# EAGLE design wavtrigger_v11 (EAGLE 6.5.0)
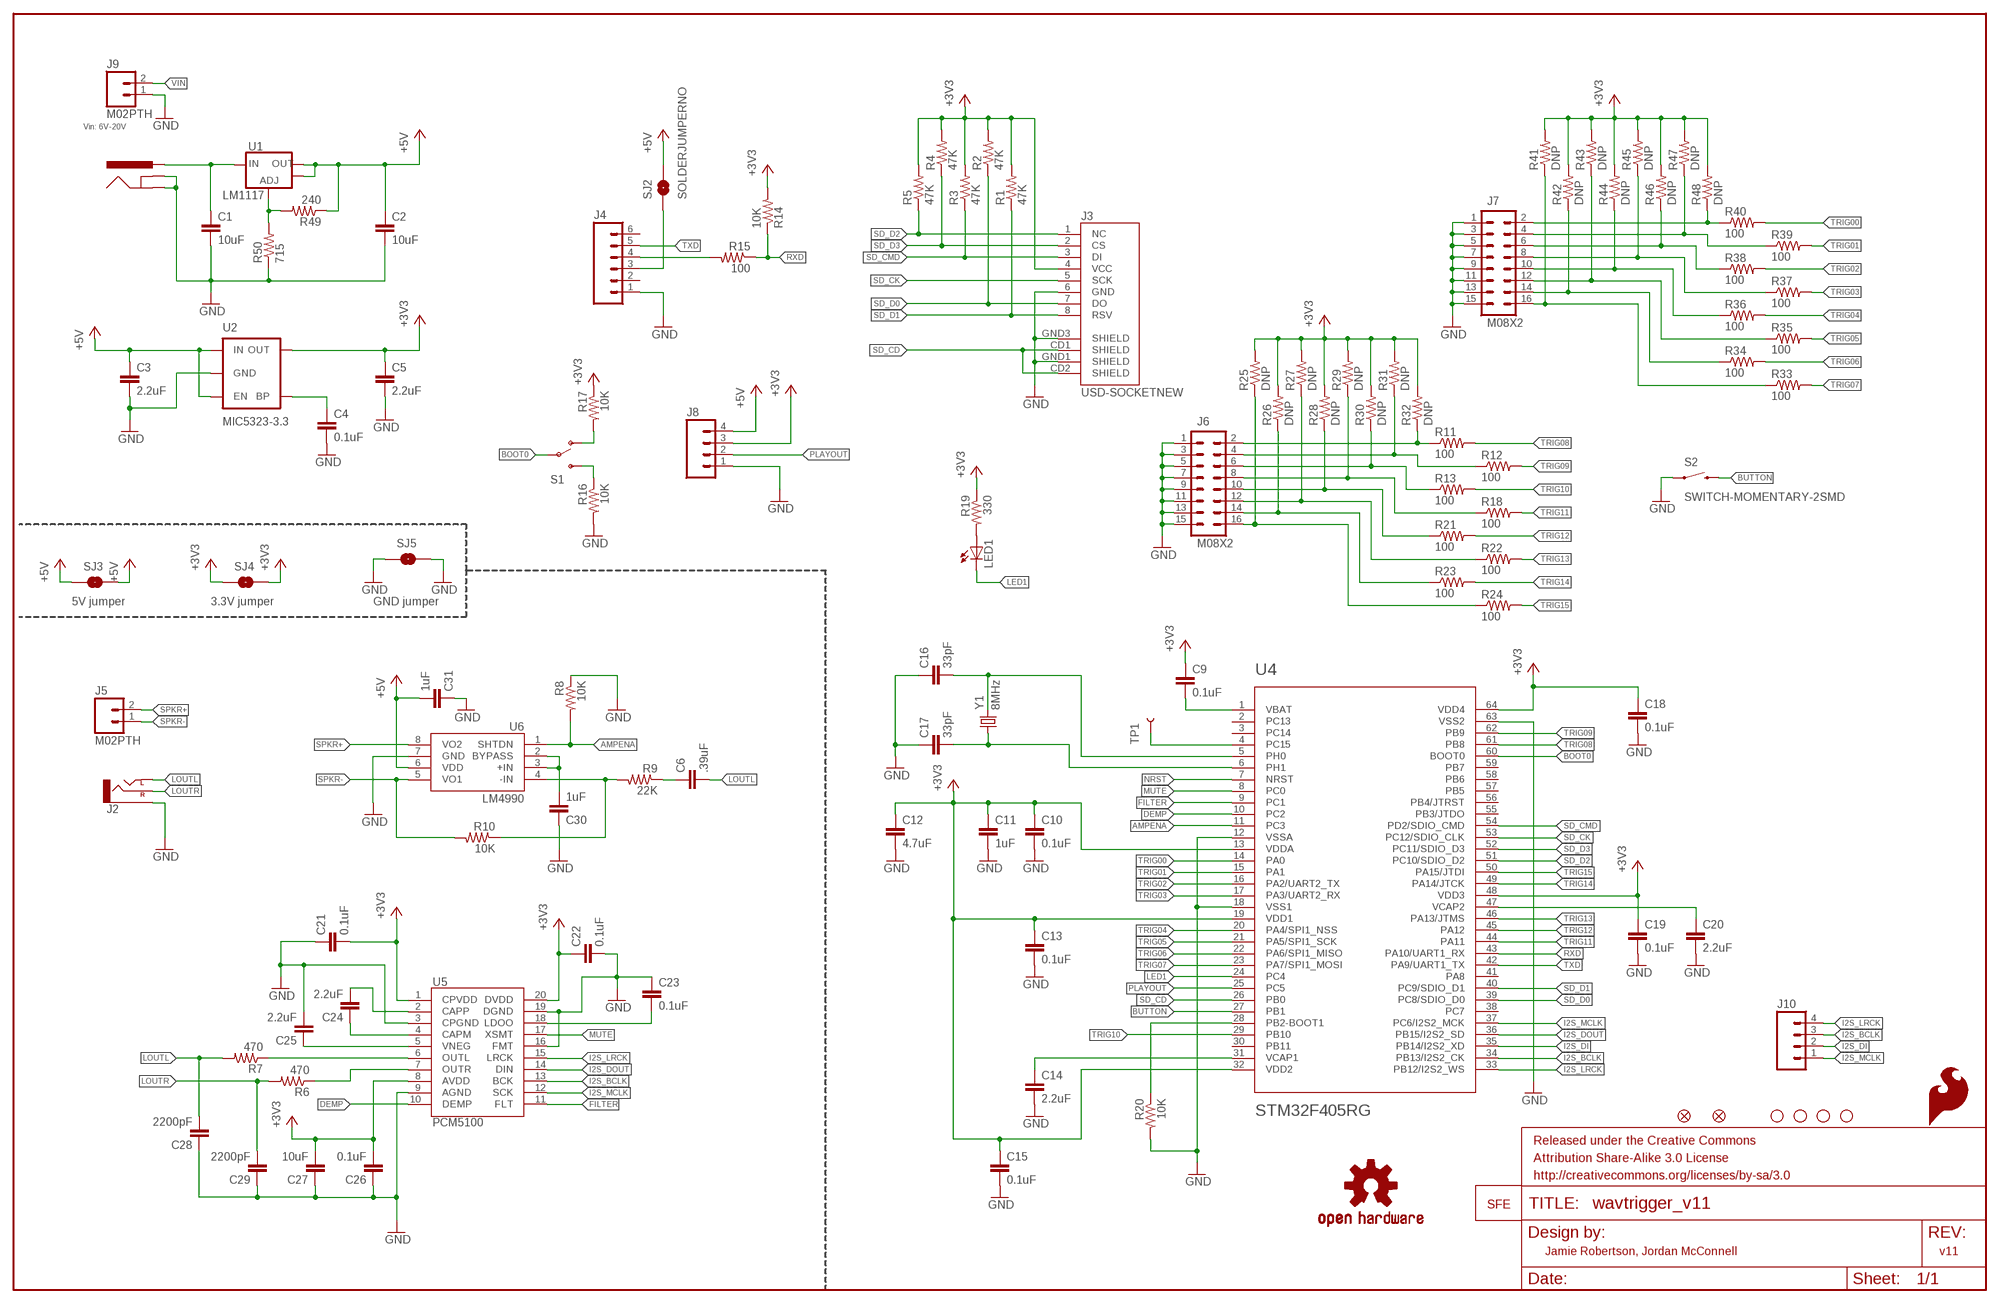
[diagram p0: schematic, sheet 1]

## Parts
C1  10uF  10UF50V20%(1210)  [1210]
C2  10uF  1UF-25V-10%(0805)  [0805]
C3  2.2uF  1UF-25V-10%(0805)  [0805]
C4  0.1uF  CAP0603-CAP  [0603-CAP]
C5  2.2uF  1UF-25V-10%(0805)  [0805]
C6  .39uF  CAP0603-CAP  [0603-CAP]
C9  0.1uF  CAP0603-CAP  [0603-CAP]
C10  0.1uF  CAP0603-CAP  [0603-CAP]
C11  1uF  CAP0603-CAP  [0603-CAP]
C12  4.7uF  CAP0603-CAP  [0603-CAP]
C13  0.1uF  CAP0603-CAP  [0603-CAP]
C14  2.2uF  CAP0603-CAP  [0603-CAP]
C15  0.1uF  CAP0603-CAP  [0603-CAP]
C16  33pF  CAP0603-CAP  [0603-CAP]
C17  33pF  CAP0603-CAP  [0603-CAP]
C18  0.1uF  CAP0603-CAP  [0603-CAP]
C19  0.1uF  CAP0603-CAP  [0603-CAP]
C20  2.2uF  CAP0603-CAP  [0603-CAP]
C21  0.1uF  CAP0603-CAP  [0603-CAP]
C22  0.1uF  CAP0603-CAP  [0603-CAP]
C23  0.1uF  CAP0603-CAP  [0603-CAP]
C24  2.2uF  CAP0603-CAP  [0603-CAP]
C25  2.2uF  CAP0603-CAP  [0603-CAP]
C26  0.1uF  CAP0603-CAP  [0603-CAP]
C27  10uF  CAP0603-CAP  [0603-CAP]
C28  2200pF  CAP0603-CAP  [0603-CAP]
C29  2200pF  CAP0603-CAP  [0603-CAP]
C30  1uF  CAP0603-CAP  [0603-CAP]
C31  1uF  CAP0603-CAP  [0603-CAP]
FID1  FIDUCIAL1X2  [FIDUCIAL-1X2]
FID2  FIDUCIAL1X2  [FIDUCIAL-1X2]
FRAME2  FRAME-LEDGER  [CREATIVE_COMMONS]
J1  5.5x2.1mm Barrel  POWER_JACKOVERPASTE_REDBOARD_0603  [POWER_JACK_SMD_OVERPASTE_REDBOARD_0603]
J2  AUDIO-JACKSMD2  [AUDIO-JACK-3.5MM-SMD]
J3  USD-SOCKETNEW  [MICRO-SD-SOCKET-PP]
J4  M06SIP  [1X06]
J5  M02PTH  [1X02]
J6  M08X2  [2X8]
J7  M08X2  [2X8]
J8  M04PTH  [1X04]
J9  M02PTH  [1X02]
J10  M04PTH  [1X04]
LED1  LED0603  [LED-0603]
LOGO1  OSHW-LOGOL  [OSHW-LOGO-L]
LOGO2  LOGO-SFENEW  [SFE-NEW-WEBLOGO]
LOGO4  SFE_LOGO_FLAME.2_INCH  [SFE_LOGO_FLAME_.2]
R1  47K  RESISTOR0603-RES  [0603-RES]
R2  47K  RESISTOR0603-RES  [0603-RES]
R3  47K  RESISTOR0603-RES  [0603-RES]
R4  47K  RESISTOR0603-RES  [0603-RES]
R5  47K  RESISTOR0603-RES  [0603-RES]
R6  470  RESISTOR0603-RES  [0603-RES]
R7  470  RESISTOR0603-RES  [0603-RES]
R8  10K  RESISTOR0603-RES  [0603-RES]
R9  22K  RESISTOR0603-RES  [0603-RES]
R10  10K  RESISTOR0603-RES  [0603-RES]
R11  100  RESISTOR0603-RES  [0603-RES]
R12  100  RESISTOR0603-RES  [0603-RES]
R13  100  RESISTOR0603-RES  [0603-RES]
R14  10K  RESISTOR0603-RES  [0603-RES]
R15  100  RESISTOR0603-RES  [0603-RES]
R16  10K  RESISTOR0603-RES  [0603-RES]
R17  10K  RESISTOR0603-RES  [0603-RES]
R18  100  RESISTOR0603-RES  [0603-RES]
R19  330  RESISTOR0603-RES  [0603-RES]
R20  10K  RESISTOR0603-RES  [0603-RES]
R21  100  RESISTOR0603-RES  [0603-RES]
R22  100  RESISTOR0603-RES  [0603-RES]
R23  100  RESISTOR0603-RES  [0603-RES]
R24  100  RESISTOR0603-RES  [0603-RES]
R25  DNP  RESISTOR0603-RES  [0603-RES]
R26  DNP  RESISTOR0603-RES  [0603-RES]
R27  DNP  RESISTOR0603-RES  [0603-RES]
R28  DNP  RESISTOR0603-RES  [0603-RES]
R29  DNP  RESISTOR0603-RES  [0603-RES]
R30  DNP  RESISTOR0603-RES  [0603-RES]
R31  DNP  RESISTOR0603-RES  [0603-RES]
R32  DNP  RESISTOR0603-RES  [0603-RES]
R33  100  RESISTOR0603-RES  [0603-RES]
R34  100  RESISTOR0603-RES  [0603-RES]
R35  100  RESISTOR0603-RES  [0603-RES]
R36  100  RESISTOR0603-RES  [0603-RES]
R37  100  RESISTOR0603-RES  [0603-RES]
R38  100  RESISTOR0603-RES  [0603-RES]
R39  100  RESISTOR0603-RES  [0603-RES]
R40  100  RESISTOR0603-RES  [0603-RES]
R41  DNP  RESISTOR0603-RES  [0603-RES]
R42  DNP  RESISTOR0603-RES  [0603-RES]
R43  DNP  RESISTOR0603-RES  [0603-RES]
R44  DNP  RESISTOR0603-RES  [0603-RES]
R45  DNP  RESISTOR0603-RES  [0603-RES]
R46  DNP  RESISTOR0603-RES  [0603-RES]
R47  DNP  RESISTOR0603-RES  [0603-RES]
R48  DNP  RESISTOR0603-RES  [0603-RES]
R49  240  240OHM1/10W1%(0603)  [0603-RES]
R50  715  RESISTOR0603  [0603-RES]
S1  SWITCH-SPDT-SMD-A  [SWITCH-SPST-SMD-A]
S2  SWITCH-MOMENTARY-2SMD  [TACTILE_SWITCH_SMD]
SJ2  SOLDERJUMPERNO  [SJ_2S-NO]
SJ3  SOLDERJUMPERTRACE  [SJ_2S-TRACE]
SJ4  SOLDERJUMPERTRACE  [SJ_2S-TRACE]
SJ5  SOLDERJUMPERTRACE  [SJ_2S-TRACE]
STANDOFF1  STAND-OFF  [STAND-OFF]
STANDOFF2  STAND-OFF  [STAND-OFF]
STANDOFF3  STAND-OFF  [STAND-OFF]
STANDOFF4  STAND-OFF  [STAND-OFF]
TP1  TEST-POINTTP_15TH_THRU  [TP_15TH]
U1  V_REG_LM1117SOT223  [SOT223]
U2  MIC5323-3.3  MIC52053.3V  [SOT23-5]
U4  STM32F405RG  [TQFP64]
U5  PCM5100  [PW_R-PDSO-G20]
U6  LM4990  [S-PDSO-G08]
Y1  8MHz  CRYSTALSMD  [HC49UP]

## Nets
+5V: C2.1 C3.1 C31.2 J8.4 R49.1 SJ2.2 SJ3.1 SJ3.2 U1.2(OUT) U1.4(OUT) U2.1(IN) U2.3(EN) U6.6(VDD)
AMPENA: R8.2 U4.11(PC3) U6.1(SHTDN)
BOOT0: S1.2(P) U4.60(BOOT0)
BUTTON: S2.3 U4.27(PB1)
DEMP: U4.10(PC2) U5.10(DEMP)
FILTER: U4.9(PC1) U5.11(FLT)
GND: C1.2 C2.2 C3.2 C4.2 C5.2 C10.2 C11.2 C12.2 C13.2 C14.2 C15.2 C16.1 C17.1 C18.2 C19.2 C20.2 C21.1 C22.2 C23.1 C25.2 C26.1 C27.1 C28.1 C29.1 C30.1 C31.1 J1.GND(GNDBREAK) J1.P$4(GND) J2.SLEEVE J3.6(GND) J3.GND1(SHIELD) J3.GND3(SHIELD) J4.1 J6.1 J6.3 J6.5 J6.7 J6.9 J6.11 J6.13 J6.15 J7.1 J7.3 J7.5 J7.7 J7.9 J7.11 J7.13 J7.15 J8.1 J9.1 R8.1 R16.2 R20.2 R50.1 S2.1 SJ5.1 SJ5.2 U2.2(GND) U4.12(VSSA) U4.18(VSS1) U4.63(VSS2) U5.3(CPGND) U5.9(AGND) U5.16(FMT) U5.19(DGND) U6.7(GND)
I2S_BCLK: J10.3 U4.34(PB13/I2S2_CK) U5.13(BCK)
I2S_DI: J10.2 U4.35(PB14/I2S2_XD)
I2S_DOUT: U4.36(PB15/I2S2_SD) U5.14(DIN)
I2S_LRCK: J10.4 U4.33(PB12/I2S2_WS) U5.15(LRCK)
I2S_MCLK: J10.1 U4.37(PC6/I2S2_MCK) U5.12(SCK)
LED1: LED1.C U4.24(PC4)
LOUTL: C6.2 C28.2 J2.TIP(LEFT) R7.2
LOUTR: C29.2 J2.RING(RIGHT) R6.2
MUTE: U4.8(PC0) U5.17(XSMT)
N$1: J6.2 R11.1 R32.1
N$2: C4.1 U2.4(BP)
N$3: C9.2 U4.1(VBAT)
N$4: C14.1 U4.31(VCAP1)
N$5: C16.2 U4.5(PH0) Y1.2
N$6: C17.2 U4.6(PH1) Y1.1
N$7: R16.1 S1.3(S)
N$8: C20.1 U4.47(VCAP2)
N$9: J4.4 R15.2
N$10: R17.2 S1.1(O)
N$11: LED1.A R19.2
N$12: R20.1 U4.28(PB2-BOOT1)
N$13: R49.2 R50.2 U1.1(ADJ)
N$14: C23.2 U5.18(LDOO)
N$15: R6.1 U5.7(OUTR)
N$16: C24.2 U5.2(CAPP)
N$17: C24.1 U5.4(CAPM)
N$18: C25.1 U5.5(VNEG)
N$19: R7.1 U5.6(OUTL)
N$20: C30.2 U6.2(BYPASS) U6.3(+IN)
N$21: C6.1 R9.1
N$22: TP1.P$1 U4.4(PC15)
N$23: J6.4 R12.1 R31.1
N$24: J6.6 R13.1 R30.1
N$25: J6.8 R18.1 R29.1
N$26: J6.10 R21.1 R28.1
N$27: J6.12 R22.1 R27.1
N$28: J6.14 R23.1 R26.1
N$29: R9.2 R10.1 U6.4(-IN)
N$30: J6.16 R24.1 R25.1
N$32: J4.3 SJ2.1
N$35: J7.2 R40.1 R48.1
N$36: J7.4 R39.1 R47.1
N$37: J7.6 R38.1 R46.1
N$38: J7.8 R37.1 R45.1
N$39: J7.10 R36.1 R44.1
N$40: J7.12 R35.1 R43.1
N$41: J7.14 R34.1 R42.1
N$42: J7.16 R33.1 R41.1
NRST: U4.7(NRST)
PLAYOUT: J8.2 U4.25(PC5)
RXD: R14.1 R15.1 U4.43(PA10/UART1_RX)
SD_CD: J3.CD1(SHIELD) J3.CD2(SHIELD) U4.26(PB0)
SD_CK: J3.5(SCK) U4.53(PC12/SDIO_CLK)
SD_CMD: J3.3(DI) R3.1 U4.54(PD2/SDIO_CMD)
SD_D0: J3.7(DO) R2.1 U4.39(PC8/SDIO_D0)
SD_D1: J3.8(RSV) R1.1 U4.40(PC9/SDIO_D1)
SD_D2: J3.1(NC) R5.1 U4.51(PC10/SDIO_D2)
SD_D3: J3.2(CS) R4.1 U4.52(PC11/SDIO_D3)
SPKR+: J5.2 U6.8(VO2)
SPKR-: J5.1 R10.2 U6.5(VO1)
TRIG00: R40.2 U4.14(PA0)
TRIG01: R39.2 U4.15(PA1)
TRIG02: R38.2 U4.16(PA2/UART2_TX)
TRIG03: R37.2 U4.17(PA3/UART2_RX)
TRIG04: R36.2 U4.20(PA4/SPI1_NSS)
TRIG05: R35.2 U4.21(PA5/SPI1_SCK)
TRIG06: R34.2 U4.22(PA6/SPI1_MISO)
TRIG07: R33.2 U4.23(PA7/SPI1_MOSI)
TRIG08: R11.2 U4.61(PB8)
TRIG09: R12.2 U4.62(PB9)
TRIG10: R13.2 U4.29(PB10)
TRIG11: R18.2 U4.44(PA11)
TRIG12: R21.2 U4.45(PA12)
TRIG13: R22.2 U4.46(PA13/JTMS)
TRIG14: R23.2 U4.49(PA14/JTCK)
TRIG15: R24.2 U4.50(PA15/JTDI)
TXD: J4.5 U4.42(PA9/UART1_TX)
VCC: C5.1 C9.1 C10.1 C11.1 C12.1 C13.1 C15.1 C18.1 C19.1 C21.2 C22.1 C26.2 C27.2 J3.4(VCC) J8.3 R1.2 R2.2 R3.2 R4.2 R5.2 R14.2 R17.1 R19.1 R25.2 R26.2 R27.2 R28.2 R29.2 R30.2 R31.2 R32.2 R41.2 R42.2 R43.2 R44.2 R45.2 R46.2 R47.2 R48.2 SJ4.1 SJ4.2 U2.5(OUT) U4.13(VDDA) U4.19(VDD1) U4.32(VDD2) U4.48(VDD3) U4.64(VDD4) U5.1(CPVDD) U5.8(AVDD) U5.20(DVDD) ; supply symbol labelled +3V3
VIN: C1.1 J1.VIN0(PWR) J9.2 U1.3(IN)
Unconnected: J4.2 J4.6 U4.2(PC13) U4.3(PC14) U4.30(PB11) U4.38(PC7) U4.41(PA8) U4.55(PB3/JTDO) U4.56(PB4/JTRST) U4.57(PB5) U4.58(PB6) U4.59(PB7)

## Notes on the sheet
- Vin: 6V-20V
- LM1117
- 5V jumper | 3.3V jumper | GND jumper
- Jamie Robertson, Jordan McConnell | v11

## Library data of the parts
C1 = SparkFun-Capacitors:10UF50V20%(1210): CAP-09824; PROD_ID: CAP-09824
C2 C3 C5 = SparkFun-Capacitors:1UF-25V-10%(0805): CAP-08064; PROD_ID: CAP-08064; VALUE: 1uF
C4 C6 C9-C31 = SparkFun-Capacitors:CAP: Capacitor
FID1 FID2 = SparkFun-Aesthetics:FIDUCIAL: Fiducial Alignment Points
FRAME2 = SparkFun-Aesthetics:FRAME-LEDGER: Schematic Frame
J1 = Testing:POWER_JACK: Power Jack This is the standard 5.5mm barrel jack for power. The PTH is the most common, proven, reliable, footprint. All others are experimental. The Slot footprint only works if the mill layer is transmitted to the PCB fab house so be warned. Spark Fun Electronics SKU : PRT-00119. Mating wall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
J2 = SparkFun-Connectors:AUDIO-JACK: 3.5mm Audio Jack Simple 3.5mm common PCB mount audio jack. SKU: PRT-08032
J3 = robertsonics:USD-SOCKET: microSD Socket Push-push type uSD socket. Schematic element and footprint production proven. Spark Fun Electronics SKU : PRT-00127. tDoc lines correctly indicate media card edge positions when inserting (unlocked, locked, depressed).
J4 = SparkFun-Connectors:M06: Header 6 Standard 6-pin 0.1" header. Use with straight break away headers (SKU : PRT-00116), right angle break away headers (PRT-00553), swiss pins (PRT-00743), machine pins (PRT-00117), and female headers (PRT-00115). Molex polarized connector foot print use with SKU : PRT-08094 with associated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
J5 J9 = SparkFun-Connectors:M02: Standard 2-pin 0.1" header. Use with
J6 J7 = SparkFun-Connectors:M08X2: .1" headers, two rows of 8 each
J8 J10 = SparkFun-Connectors:M04: Header 4 Standard 4-pin 0.1" header. Use with straight break away headers (SKU : PRT-00116), right angle break away headers (PRT-00553), swiss pins (PRT-00743), machine pins (PRT-00117), and female headers (PRT-00115). Molex polarized connector foot print use with SKU : PRT-08231 with associated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
LED1 = SparkFun-LED:LED: LEDs
LOGO1 = SparkFun-Aesthetics:OSHW-LOGO: Open Source Hardware Logo This logo indicates the piece of hardware it is found on incorporates a OSHW license and/or adheres to the definition of open source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
LOGO2 = SparkFun-Aesthetics:LOGO-SFE: Spark Fun Electronics PCB Logo
LOGO4 = SparkFun-Aesthetics:SFE_LOGO_FLAME: SFE Logo, flame only
R1-R48 = SparkFun-Passives:RESISTOR: Resistor
R49 = SparkFun-Resistors:240OHM1/10W1%(0603): RES-07849; PROD_ID: RES-07849
R50 = SparkFun-Resistors:RESISTOR: Resistor
S1 = SparkFun-Electromechanical:SWITCH-SPDT: SPDT Switch Simple slide switch, Spark Fun Electronics SKU : COM-00102 DPDT SMT slide switch, AYZ0202, SWCH-08179
S2 = SparkFun-Electromechanical:SWITCH-MOMENTARY-2: Various NO switches- pushbuttons, reed, etc
SJ2-SJ5 = SparkFun-Passives:SOLDERJUMPER: Solder Jumper
STANDOFF1-STANDOFF4 = SparkFun-Electromechanical:STAND-OFF: #4 Stand Off
TP1 = SparkFun-Passives:TEST-POINT: Bare copper test points for troubleshooting or ICT
U1 = SparkFun-PowerIC:V_REG_LM1117: Voltage Regulator LM1117 Standard adjustable voltage regulator but in SMD form. Spark Fun Electronics SKU : COM-00595
U2 = SparkFun-PowerIC:MIC5205: MIC5205 150mA vreg 3.3V - VREG-00822 5V - VREG-00823; PROD_ID: VREG-00822
U4 = SparkFun-DigitalIC:STM32F405RG: ARM DSP Chip used on the WAV Trigger board.
U5 = robertsonics:PCM5100: PCM5100 Stereo DAC
U6 = robertsonics:LM4990: LM4990 2 Watt Audio Amp
Y1 = SparkFun-FreqCtrl:CRYSTAL: Various standard crystals. Proven footprints. Spark Fun Electronics SKU : COM-00534

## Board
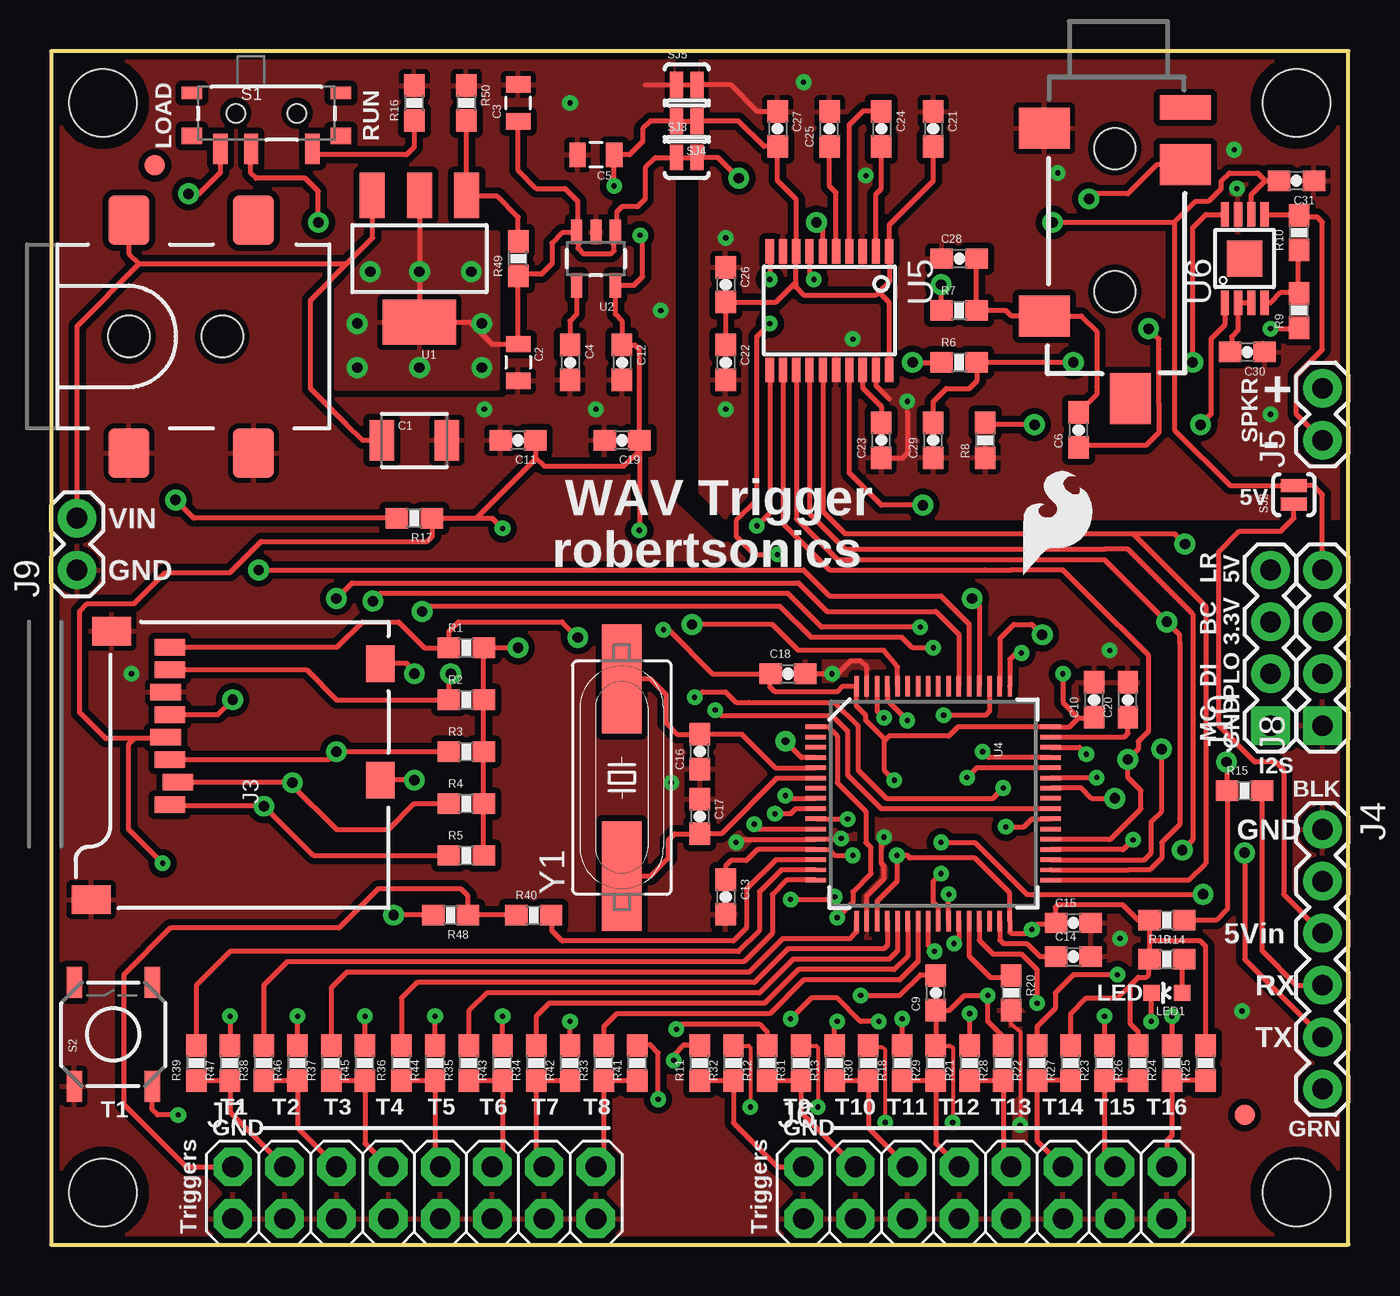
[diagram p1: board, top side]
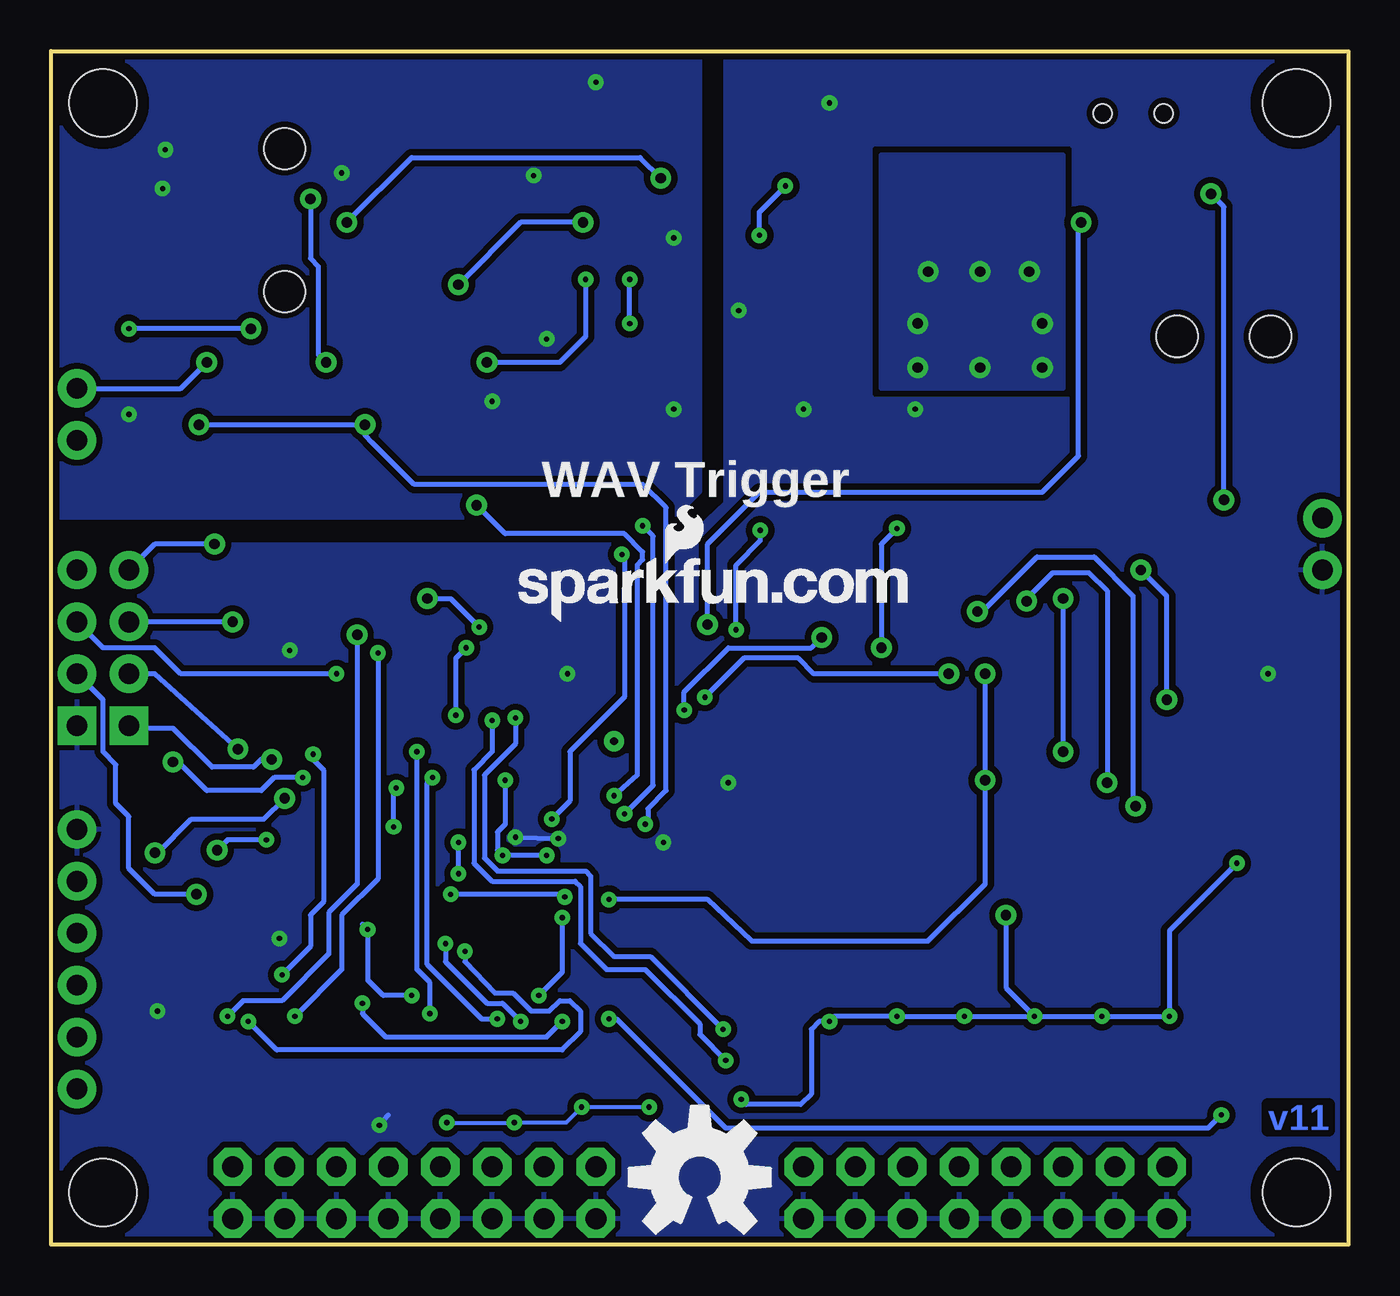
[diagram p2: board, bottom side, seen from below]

Size 63.5 x 58.42 mm. Coordinates in mm from the lower left corner, seen from the top.
Outline: 0,0 63.5,0 63.5,58.42 0,58.41 0,0
Copper layers (1*16): Top 0.035mm / dielectric 1.5mm / Bottom 0.035mm
Design rules "SparkFun": minimum track width 8mil, minimum drill 20mil, track to track 8mil, track to pad 8mil, pad to pad 8mil, via to via 8mil, smd to smd 8mil, copper to edge 8mil, drill to drill 8mil, minimum pad ring 12mil, minimum via ring 10mil, stop-mask expansion 4mil, vias tented up to drill 20mil, thermal gap 10mil

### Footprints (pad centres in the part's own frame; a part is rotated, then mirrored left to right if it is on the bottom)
1210 = smd 1.2 x 2: 1 -1.6,0; 2 1.6,0
0805 = smd 0.8 x 1.2: 1 -0.9,0; 2 0.9,0
0603-CAP = smd 1.1 x 1: 1 -0.85,0; 2 0.85,0
FIDUCIAL-1X2 = smd 1 x 1: 1 0,0
POWER_JACK_SMD_OVERPASTE_REDBOARD_0603 = smd 2 x 2.4: GND 0,-5.7; P$4 6.1,-5.7; VIN0 0,5.7; VIN1 6.1,5.7 | hole 2.032: 0,0; 4.572,0
AUDIO-JACK-3.5MM-SMD = smd 2 x 2.5: RING 4.3,3.45; SLEEVE 2.5,-3.45; TIP 11.7,-3.45 | smd 1.2 x 2.5: RSH 1.5,3.45 | smd 2.5 x 2: TSH 15.75,0.75 | hole 2: 3.5,0; 10.5,0
MICRO-SD-SOCKET-PP = smd 0.8 x 1.5: 1 -8.94,10.7; 2 -7.84,10.3; 3 -6.74,10.7; 4 -5.64,10.9; 5 -4.54,10.7; 6 -3.44,10.9; 7 -2.34,10.7; 8 -1.24,10.7 | smd 1.8 x 1.4: CD1 -2.05,0.4; CD2 -7.75,0.4 | smd 1.4 x 1.9: GND1 -13.6,14.55; GND3 -0.45,13.55
1X06 = drill 1.016 pad 1.88: 1 0,0; 2 2.54,0; 3 5.08,0; 4 7.62,0; 5 10.16,0; 6 12.7,0
1X02 = drill 1.016 pad 1.88: 1 0,0; 2 2.54,0
2X8 = drill 1.016 pad 1.88 octagon: 1 0,0; 2 0,2.54; 3 2.54,0; 4 2.54,2.54; 5 5.08,0; 6 5.08,2.54; 7 7.62,0; 8 7.62,2.54; 9 10.16,0; 10 10.16,2.54; 11 12.7,0; 12 12.7,2.54; 13 15.24,0; 14 15.24,2.54; 15 17.78,0; 16 17.78,2.54
1X04 = drill 1.016 pad 1.88 square: 1 0,0 | drill 1.016 pad 1.88: 2 2.54,0; 3 5.08,0; 4 7.62,0
LED-0603 = smd 0.8 x 0.8: A 0,-0.75; C 0,0.75
0603-RES = smd 1.1 x 1: 1 -0.85,0; 2 0.85,0
SWITCH-SPST-SMD-A = smd 0.7 x 1.5: 1 -2.25,-1.75; 2 -0.75,-1.75; 3 2.25,-1.75 | smd 1 x 0.6: GND1 -3.65,1; GND3 3.65,1 | smd 1 x 0.8: GND2 -3.65,-1.1; GND4 3.65,-1.1 | hole 0.9: -1.5,0; 1.5,0
TACTILE_SWITCH_SMD = smd 1.524 x 0.762: 1 -2.54,1.905; 2 2.54,1.905; 3 -2.54,-1.905; 4 2.54,-1.905
SJ_2S-NO = smd 0.635 x 1.27: 1 -0.45,0; 2 0.45,0
SJ_2S-TRACE = smd 0.635 x 1.27: 1 -0.508,0; 2 0.508,0
STAND-OFF = hole 3.302: 0,0
TP_15TH = drill 0.381 pad 0.61: P$1 0,0
SOT223 = smd 1.219 x 2.235: 1 -2.311,-3.099; 2 0,-3.099; 3 2.311,-3.099 | smd 3.6 x 2.2: 4 0,3.099
SOT23-5 = smd 0.55 x 1.2: 1 -0.95,-1.3; 2 0,-1.3; 3 0.95,-1.3; 4 0.95,1.3; 5 -0.95,1.3
TQFP64 = smd 0.22 x 1: 1 -3.75,-5.75; 2 -3.25,-5.75; 3 -2.75,-5.75; 4 -2.25,-5.75; 5 -1.75,-5.75; 6 -1.25,-5.75; 7 -0.75,-5.75; 8 -0.25,-5.75; 9 0.25,-5.75; 10 0.75,-5.75; 11 1.25,-5.75; 12 1.75,-5.75; 13 2.25,-5.75; 14 2.75,-5.75; 15 3.25,-5.75; 16 3.75,-5.75; 33 3.75,5.75; 34 3.25,5.75; 35 2.75,5.75; 36 2.25,5.75; 37 1.75,5.75; 38 1.25,5.75; 39 0.75,5.75; 40 0.25,5.75; 41 -0.25,5.75; 42 -0.75,5.75; 43 -1.25,5.75; 44 -1.75,5.75; 45 -2.25,5.75; 46 -2.75,5.75; 47 -3.25,5.75; 48 -3.75,5.75 | smd 1 x 0.22: 17 5.75,-3.75; 18 5.75,-3.25; 19 5.75,-2.75; 20 5.75,-2.25; 21 5.75,-1.75; 22 5.75,-1.25; 23 5.75,-0.75; 24 5.75,-0.25; 25 5.75,0.25; 26 5.75,0.75; 27 5.75,1.25; 28 5.75,1.75; 29 5.75,2.25; 30 5.75,2.75; 31 5.75,3.25; 32 5.75,3.75; 49 -5.75,3.75; 50 -5.75,3.25; 51 -5.75,2.75; 52 -5.75,2.25; 53 -5.75,1.75; 54 -5.75,1.25; 55 -5.75,0.75; 56 -5.75,0.25; 57 -5.75,-0.25; 58 -5.75,-0.75; 59 -5.75,-1.25; 60 -5.75,-1.75; 61 -5.75,-2.25; 62 -5.75,-2.75; 63 -5.75,-3.25; 64 -5.75,-3.75
PW_R-PDSO-G20 = smd 0.4 x 1.2: 1 -2.925,-2.9; 2 -2.275,-2.9; 3 -1.625,-2.9; 4 -0.975,-2.9; 5 -0.325,-2.9; 6 0.325,-2.9; 7 0.975,-2.9; 8 1.625,-2.9; 9 2.275,-2.9; 10 2.925,-2.9; 11 2.925,2.9; 12 2.275,2.9; 13 1.625,2.9; 14 0.975,2.9; 15 0.325,2.9; 16 -0.325,2.9; 17 -0.975,2.9; 18 -1.625,2.9; 19 -2.275,2.9; 20 -2.925,2.9
S-PDSO-G08 = smd 0.4 x 1.2: 1 -0.975,-2.157; 2 -0.325,-2.157; 3 0.325,-2.157; 4 0.975,-2.157; 5 0.975,2.157; 6 0.325,2.157; 7 -0.325,2.157; 8 -0.975,2.157 | smd 1.73 x 1.78: TH 0,0
HC49UP = smd 5.334 x 1.93: 1 -4.826,0; 2 4.826,0

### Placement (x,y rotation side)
C1  17.78,39.37 0 top
C2  22.86,43.18 270 top
C3  22.86,55.88 90 top
C4  25.4,43.18 270 top
C5  26.67,53.34 180 top
C6  50.29,39.88 90 top
C9  43.31,12.32 90 top
C10  51.05,26.67 90 top
C11  22.86,39.37 180 top
C12  27.94,43.18 270 top
C13  33.02,17.02 270 top
C14  50.04,14.1 0 top
C15  50.04,15.75 0 top
C16  31.75,24.13 90 top
C17  31.75,20.95 270 top
C18  36.07,27.94 0 top
C19  27.94,39.37 180 top
C20  52.7,26.67 90 top
C21  43.18,54.61 270 top
C22  33.02,43.18 270 top
C23  40.64,39.37 90 top
C24  40.64,54.61 270 top
C25  38.1,54.61 90 top
C26  33.02,46.99 270 top
C27  35.56,54.61 270 top
C28  44.45,48.26 0 top
C29  43.18,39.37 90 top
C30  58.55,43.69 180 top
C31  60.96,52.07 180 top
FID1  5.08,52.83 0 top
FID2  58.42,6.35 0 top
FRAME2  not placed on the board
J1  3.81,44.45 0 top
J2  52.07,57.15 270 top
J3  16.51,30.48 90 top
J4  62.23,20.32 270 top
J5  62.23,39.37 90 top
J6  36.83,1.27 0 top
J7  8.89,1.27 0 top
J8  62.23,25.4 90 top
J9  1.27,33.02 90 top
J10  59.69,25.4 90 top
LED1  54.61,12.32 90 top
LOGO1  31.75,3.3 0 bottom
LOGO2  40.64,30.48 0 bottom
LOGO4  47.24,32.51 0 top
R1  20.32,29.21 0 top
R2  20.32,26.67 0 top
R3  20.32,24.13 0 top
R4  20.32,21.59 0 top
R5  20.32,19.05 0 top
R6  44.45,43.18 0 top
R7  44.45,45.72 0 top
R8  45.72,39.37 90 top
R9  61.09,45.72 90 top
R10  61.09,49.53 90 top
R11  31.75,8.89 90 top
R12  35.05,8.89 90 top
R13  38.35,8.89 90 top
R14  54.61,15.88 180 top
R15  58.42,22.23 0 top
R16  17.78,55.88 90 top
R17  17.78,35.56 180 top
R18  41.66,8.89 90 top
R19  54.61,13.97 0 top
R20  46.99,12.32 270 top
R21  44.96,8.89 90 top
R22  48.26,8.89 90 top
R23  51.56,8.89 90 top
R24  54.86,8.89 90 top
R25  56.52,8.89 90 top
R26  53.21,8.89 90 top
R27  49.91,8.89 90 top
R28  46.61,8.89 90 top
R29  43.31,8.89 90 top
R30  40.01,8.89 90 top
R31  36.7,8.89 90 top
R32  33.4,8.89 90 top
R33  27.05,8.89 90 top
R34  23.75,8.89 90 top
R35  20.45,8.89 90 top
R36  17.14,8.89 90 top
R37  13.72,8.89 90 top
R38  10.41,8.89 90 top
R39  7.11,8.89 90 top
R40  23.62,16.13 0 top
R41  28.7,8.89 90 top
R42  25.4,8.89 90 top
R43  22.1,8.89 90 top
R44  18.8,8.89 90 top
R45  15.37,8.89 90 top
R46  12.06,8.89 90 top
R47  8.76,8.89 90 top
R48  19.56,16.13 180 top
R49  22.86,48.26 90 top
R50  20.32,55.88 270 top
S1  10.54,55.37 0 top
S2  3.05,10.29 90 top
SJ2  60.83,36.7 90 top
SJ3  31.11,53.21 0 top
SJ4  31.11,54.99 180 top
SJ5  31.11,56.77 0 top
STANDOFF1  2.54,2.54 0 top
STANDOFF2  60.96,2.54 0 top
STANDOFF3  2.54,55.88 0 top
STANDOFF4  60.96,55.88 0 top
TP1  35.94,24.64 0 top
U1  18.03,48.26 180 top
U2  26.67,48.26 180 top
U4  43.18,21.59 270 top
U5  38.1,45.72 180 top
U6  58.42,48.26 0 top
Y1  27.94,22.86 90 top

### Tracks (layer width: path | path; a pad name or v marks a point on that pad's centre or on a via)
+5V  (via drill 0.51)
  Top 0.254: U6.6 58.74,51.38 59.44,52.07 | 54.99,50.04 56.01,51.05 56.64,51.05 57.28,51.69 57.28,52.07 57.66,52.45 59.05,52.45 59.44,52.07 | 54.99,50.04 54.99,39.88 57.72,37.15 SJ2.2 | v49.02,50.04 54.99,50.04 | 25.78,49.62 U2.3 25.69,49.53 25.02,49.53 24.51,49.02 24.51,48.01 24,47.5 22.95,47.5 R49.1 C2.1 21.59,44.07 20.5,45.16 U1.4 v18.03,47.62 U1.2 | 25.78,49.62 25.78,51.05 25.15,51.69 23.75,51.69 22.86,52.58 C3.1 | 25.78,49.62 25.78,48.77 26.04,48.51 27.43,48.51 27.56,48.64 27.56,49.5 U2.1 27.69,49.63 27.69,50.55 27.94,50.8 28.7,50.8 29.08,51.18 29.08,52.7 29.59,53.21 SJ3.1 SJ3.2 32.64,53.21 v33.66,52.2 | 60.76,37.08 SJ2.2 | J8.4 62.23,36.7 61.78,37.15 SJ2.2 | 60.89,37.21 SJ2.2 | 59.44,52.07 C31.2
  Bottom 0.254: v49.02,50.04 45.85,53.21 34.67,53.21 v33.66,52.2
  other vias: 15.62,47.62 20.57,47.62 14.99,42.93 18.03,42.93 21.08,42.93 14.99,45.09 21.08,45.09
  pour Top (isolate 0.305): 13.97,49.53 21.84,49.53 21.84,41.91 13.97,41.91
  pour Bottom (isolate 0.305): 13.97,41.91 22.86,41.91 22.86,53.34 13.97,53.34
AMPENA  (via drill 0.25, 0.51)
  Top 0.254: U6.1 57.45,45 56.77,44.32 56.77,40.64 v56.26,40.13 | v34.42,20.57 34.65,20.34 U4.11 | v48.13,40.13 45.81,40.13 R8.2
  Bottom 0.254: v34.42,20.57 34.29,20.7 34.29,21.34 33.4,22.23 33.4,36.07 34.54,37.21 44.83,37.21 45.72,37.21 47.75,39.24 48.13,39.62 v48.13,40.13 v56.26,40.13
BOOT0  (via drill 0.51)
  Top 0.254: v31.37,30.35 35.31,30.35 36.58,29.08 40.77,29.08 41.43,28.29 U4.60 | S1.2 9.78,52.45 10.03,52.2 12.45,52.2 13.08,51.56 v13.08,50.04
  Bottom 0.254: v31.37,30.35 31.37,34.29 28.83,36.83 14.99,36.83 13.21,38.61 13.21,49.91 v13.08,50.04
BUTTON  (via drill 0.25)
  Top 0.254: U4.27 44.43,14.97 v44.2,14.73 | v40.51,10.92 39.62,10.92 38.48,12.06 37.21,12.06 v36.2,11.05 | v6.22,6.35 5.21,6.35 4.95,6.6 S2.3
  Bottom 0.254: v44.2,14.73 44.2,13.84 42.16,11.81 41.4,11.81 v40.51,10.92 | v36.2,11.05 35.81,11.05 30.48,5.71 6.86,5.71 v6.22,6.35
DEMP  (via drill 0.25)
  Top 0.254: U5.10 v35.17,47.25 v35.18,47.24 | v35.18,45.09 34.54,44.45 34.54,36.45 33.53,35.43 33.53,34.67 34.42,33.78 v35.56,33.78 | U4.10 38.98,20.84 v38.99,20.83
  Bottom 0.254: v35.18,45.09 v35.18,47.24 | v35.56,33.78 35.43,33.66 35.43,26.8 38.1,24.13 38.1,21.72 v38.99,20.83
FILTER  (via drill 0.25)
  Top 0.254: U5.11 35.17,35.81 v34.54,35.18 | v35.43,21.08 36.2,21.08 36.45,21.34 U4.9
  Bottom 0.254: v35.43,21.08 34.04,22.48 34.04,34.67 v34.54,35.18
GND  (via drill 0.25)
  Top 0.203: R20.2 46.99,10.79 47.43,10.41 v47.43,5.84
  Top 0.254: C27.1 34.58,55.46 33.27,56.77 SJ5.2 SJ5.1 29.08,56.77 | U4.63 39.93,28.27 39.62,28.57 39.12,28.57 38.48,27.94 C18.2 | U4.18 39.93,17.07 40.77,17.91 40.77,18.54 40.64,18.67 40.64,19.81 v40.77,19.94 | U5.19 40.38,42.05 41.02,41.4 | 41.91,40.77 41.91,38.73 41.66,38.48 40.68,38.48 C23.1 | v33.53,19.68 33.68,19.84 U4.12 38.64,19.84 v38.67,19.88
  Bottom 0.254: v47.43,5.84 46.99,6.35 | v40.77,19.94 v38.67,19.88
  other vias: 30.35,22.61 58.04,51.69 57.91,53.59 59.69,40.64 39.88,52.32 33.02,49.28 33.02,40.89 41.91,41.27 51.82,29.08 58.29,11.43 52.32,14.99 38.23,27.94 3.94,27.94 29.84,45.72 39.24,44.32 26.67,40.89 21.21,40.89 25.4,55.88 36.83,56.9 49.28,52.45
  pour Bottom (isolate 0.305, rank 2): 0,58.42 0,0 63.5,0 63.5,34.29 32.64,34.29 30.48,36.32 30.48,58.42
  pour Top (isolate 0.305, rank 2): 0,58.42 0,0 63.5,0 63.5,34.29 32.64,34.29 30.48,36.32 30.48,58.42
  pour Top (isolate 0.305): 31.75,58.42 31.75,36.83 33.02,35.56 63.5,35.56 63.5,58.42
  pour Bottom (isolate 0.305): 31.75,58.42 31.75,36.83 33.02,35.56 63.5,35.56 63.5,58.42
I2S_BCLK  (via drill 0.51)
  Top 0.254: U5.13 36.48,35.53 38.48,33.53 51.18,33.53 51.56,33.53 v54.61,30.48 55.24,29.84 55.24,29.46 55.24,20.83 55.24,20.57 54.36,19.68 54.36,18.92 53.77,18.34 52.76,18.34 U4.34
  Bottom 0.254: v54.61,30.48 J10.3
I2S_DI  (via drill 0.51)
  Top 0.254: U4.35 53.51,18.84 53.85,19.18 53.85,20.7 54.36,21.21 v54.36,24.26
  Bottom 0.254: v54.36,24.26 58.42,27.94 J10.2
I2S_DOUT  (via drill 0.25, 0.51)
  Top 0.254: U5.14 37.12,35.77 38.86,34.04 51.56,34.04 52.7,34.04 55.88,30.86 55.88,19.81 v55.37,19.3 | U4.36 52.41,19.34 52.49,19.34 v52.96,19.81
  Bottom 0.254: v52.96,19.81 54.86,19.81 v55.37,19.3
I2S_LRCK  (via drill 0.51)
  Top 0.254: U5.15 37.77,35.88 38.86,34.8 52.96,34.8 | 52.96,34.8 56.52,31.24 56.52,18.67 55.69,17.84 U4.33 | 52.96,34.8 53.85,34.8 54.99,34.8 v55.5,34.29
  Bottom 0.254: v55.5,34.29 58.42,34.29 J10.4
I2S_MCLK  (via drill 0.51)
  Top 0.254: U5.12 35.83,35.3 38.1,33.02 45.72,33.02 46.99,33.02 49.53,33.02 50.8,31.75 53.72,28.83 53.72,25.15 53.21,24.64 53.21,24.26 v52.7,23.75 52.7,22.86 53.34,22.23 53.34,21.34 51.84,19.84 51.72,19.84 U4.37
  Bottom 0.254: v52.7,23.75 53.21,23.75 53.59,23.37 55.63,23.37 57.53,25.27 59.56,25.27 J10.1
LED1  (via drill 0.25)
  Top 0.254: v53.85,10.92 53.85,12.31 LED1.C | U4.24 42.93,14.66 v43.24,14.35
  Bottom 0.254: v43.24,14.35 43.24,13.84 41.78,12.32 40.89,12.32 40.01,11.43 39.12,11.43 38.61,11.94 38.1,11.94 37.59,11.43 37.59,10.41 38.48,9.53 52.45,9.53 v53.85,10.92
LOUTL
  Top 0.254: C28.2 R7.2 46.74,45.72 47.01,45.45 J2.TIP 50.44,45.45 51.18,44.7 51.18,42 51.18,41.62 C6.2
LOUTR  (via drill 0.51)
  Top 0.254: C29.2 43.18,41.27 43.81,41.91 44.96,41.91 45.34,42.29 45.34,43.14 R6.2 v50.04,43.18 | J2.RING 54.12,52.85 52.7,51.44 51.05,51.44 v50.8,51.18
  Bottom 0.254: v50.8,51.18 50.8,48.26 50.42,47.88 50.42,43.56 v50.04,43.18
MUTE  (via drill 0.25, 0.51)
  Top 0.254: 39.12,42.78 U5.17 39.08,37.76 40.64,36.2 v42.67,36.2 | v35.94,21.97 36.07,21.84 U4.8
  Bottom 0.254: v35.94,21.97 34.8,22.99 34.8,33.27 34.54,33.53 34.54,33.91 35.43,34.8 41.27,34.8 v42.67,36.2
N$1
  Top 0.254: R11.1 R32.1 33.4,5.97 35.56,3.81 J6.2
N$2
  Top 0.254: U2.4 25.72,45.53 25.4,45.21 C4.1
N$3  (via drill 0.25)
  Top 0.254: v39.62,12.19 41.53,12.19 42.55,13.21 43.27,13.21 C9.2 | v38.48,16 39.24,16.76 39.24,17.27 40.13,18.16 40.13,19.43 39.88,19.68 39.88,21.21 38.48,22.61 38.48,24.89 38.03,25.34 U4.1
  Bottom 0.254: v38.48,16 38.48,13.34 v39.62,12.19
N$4
  Top 0.254: U4.31 46.43,14.91 46.61,14.73 47.75,14.73 48.39,14.1 C14.1
N$5
  Top 0.254: Y1.2 29.34,27.69 30.1,26.92 30.1,25.53 30.65,24.98 C16.2 33.82,24.98 35.46,23.34 U4.5
N$6
  Top 0.254: Y1.1 29.34,18.03 30.23,18.92 30.23,19.81 30.52,20.11 C17.2 32.8,20.11 35.54,22.84 U4.6
N$7
  Top 0.254: R16.1 17.78,53.72 17.4,53.34 13.07,53.34 S1.3
N$8
  Top 0.254: U4.47 52.53,24.84 52.7,25.02 C20.1
N$9
  Top 0.254: R15.2 59.27,14.39 60.96,12.7 J4.4
N$10  (via drill 0.51)
  Top 0.254: R17.2 6.99,35.56 v6.1,36.45 | v6.73,51.44 7.24,51.44 8.29,52.49 S1.1
  Bottom 0.254: v6.1,36.45 6.1,50.8 v6.73,51.44
N$11
  Top 0.254: LED1.A 55.36,13.87 R19.2
N$12
  Top 0.254: U4.28 44.93,14.12 45.97,13.08 46.9,13.08 R20.1
N$13
  Top 0.254: R49.2 22.86,50.29 21.84,51.31 20.4,51.31 U1.1 20.34,55.01 R50.2
N$14
  Top 0.254: U5.18 39.73,41.94 40.64,41.02 C23.2
N$15  (via drill 0.25, 0.51)
  Top 0.254: U5.7 37.12,47.46 v37.34,47.24 | v42.16,43.18 R6.1
  Bottom 0.254: v37.34,47.24 37.34,44.45 38.61,43.18 v42.16,43.18
N$16
  Top 0.254: U5.2 40.38,51.42 40.64,51.69 C24.2
N$17
  Top 0.254: U5.4 39.08,54.82 39.75,55.5 40.6,55.5 C24.1
N$18
  Top 0.254: U5.5 38.42,51.49 38.1,51.82 C25.1
N$19  (via drill 0.51)
  Top 0.254: U5.6 37.77,49.73 v37.47,50.04 | v43.56,46.99 43.56,45.76 R7.1
  Bottom 0.254: v37.47,50.04 40.51,50.04 v43.56,46.99
N$20
  Top 0.254: C30.2 57.78,43.78 57.78,44.45 58.09,44.76 U6.2 U6.3
N$21  (via drill 0.25, 0.51)
  Top 0.254: v59.69,44.83 61.05,44.83 R9.1 | v53.72,44.83 54.23,44.32 54.23,43.81 54.23,41.15 54.23,39.75 53.59,39.12 51.6,39.12 50.38,39.12 C6.1
  Bottom 0.254: v53.72,44.83 v59.69,44.83
N$22
  Top 0.254: U4.4 36.74,23.84 TP1.P$1
N$23
  Top 0.254: R12.1 R31.1 36.7,6.48 J6.4
N$24
  Top 0.254: J6.6 40.01,5.71 R30.1 R13.1
N$25
  Top 0.254: J6.8 43.31,4.95 R29.1 R18.1
N$26
  Top 0.254: J6.10 46.61,4.19 R28.1 R21.1
N$27
  Top 0.254: R27.1 R22.1 48.26,5.08 J6.12
N$28
  Top 0.254: R26.1 R23.1 51.56,4.32 J6.14
N$29
  Top 0.254: U6.4 59.69,46.1 60.2,46.61 61.05,46.61 | 61.05,46.61 R9.2 | 61.05,46.61 61.05,48.64 R10.1
N$30
  Top 0.254: R25.1 R24.1 54.86,5.33 54.61,5.08 J6.16
N$32
  Top 0.254: J4.3 60.33,17.14 60.33,23.11 60.33,23.24 59.94,23.62 58.93,23.62 57.15,25.4 57.15,33.91 58.17,34.92 60.2,34.92 60.83,35.56 SJ2.1
N$35
  Top 0.254: R40.1 R48.1 20.41,17.06 20.07,17.4 16,17.4 14.1,15.49 5.84,15.49 3.56,13.21 3.56,6.86 6.6,3.81 J7.2
N$36
  Top 0.254: J7.4 8.76,6.48 R47.1 R39.1
N$37
  Top 0.254: J7.6 12.06,5.71 R46.1 R38.1
N$38
  Top 0.254: J7.8 15.37,4.95 R45.1 R37.1
N$39
  Top 0.254: J7.10 18.8,4.06 R44.1 R36.1
N$40
  Top 0.254: R35.1 R43.1 22.1,4.32 J7.12
N$41
  Top 0.254: J7.14 23.75,4.19 R34.1 R42.1
N$42
  Top 0.254: J7.16 27.05,4.19 R33.1 R41.1
PLAYOUT  (via drill 0.25, 0.51)
  Top 0.254: U4.25 43.43,16.51 43.18,16.76 43.18,17.78 v43.56,18.16 | v56.39,17.14 47.75,17.14 45.21,19.68 v43.56,19.68
  Bottom 0.254: v56.39,17.14 58.42,17.14 59.69,18.41 59.69,20.95 60.33,21.59 60.33,23.5 60.96,24.13 60.96,26.67 J8.2 | v43.56,18.16 v43.56,19.68
RXD  (via drill 0.25, 0.51)
  Top 0.254: R14.1 57.02,15.88 57.57,16.42 R15.1 57.57,23.58 v57.53,23.62 | v51.18,22.86 51.16,22.84 U4.43
  Bottom 0.254: v57.53,23.62 57.28,23.62 56.52,22.86 55.88,22.23 53.21,22.23 52.58,22.86 v51.18,22.86
SD_CD  (via drill 0.25, 0.51)
  Top 0.254: v17.78,27.94 17.78,28.07 17.4,28.45 16.13,28.45 J3.CD1 | v36.2,16.89 38.23,16.89 v38.35,17.02 | U4.26 43.93,17.01 v43.94,17.14 | v17.78,22.73 J3.CD2
  Bottom 0.254: v36.2,16.89 31.37,16.89 29.21,14.86 20.57,14.86 17.78,17.65 v17.78,22.73 v17.78,27.94 | v38.35,17.02 38.48,17.14 v43.94,17.14
SD_CK  (via drill 0.51)
  Top 0.254: J3.5 8.16,25.94 v8.89,26.67 | v10.16,33.02 36.83,33.02 38.1,31.75 43.56,31.75 44.93,30.38 U4.53
  Bottom 0.254: v8.89,26.67 8.89,31.75 v10.16,33.02
SD_CMD  (via drill 0.51)
  Top 0.254: J3.3 13.58,23.74 v13.97,24.13 R3.1 | v13.97,31.62 14.73,32.38 36.58,32.38 37.97,30.99 43.31,30.99 44.43,29.86 U4.54
  Bottom 0.254: v13.97,31.62 v13.97,24.13
SD_D0  (via drill 0.25, 0.51)
  Top 0.254: J3.7 12.5,28.14 13.97,26.67 R2.1 19.47,27.85 v19.56,27.94 | v46.74,20.45 47.62,20.45 48.02,20.84 U4.39 | v46.61,22.35 46.1,21.84 40.89,21.84 39.5,23.24 39.5,25.4 38.35,26.54 34.16,26.54 33.53,26.54 33.02,27.05 31.88,27.05 31.62,26.8 v31.5,26.8
  Bottom 0.254: v19.56,27.94 26.16,27.94 26.92,28.7 29.59,28.7 v31.5,26.8 | v46.74,20.45 46.74,22.23 v46.61,22.35
SD_D1  (via drill 0.25, 0.51)
  Top 0.254: J3.8 14,29.24 15.24,30.48 17.02,30.48 18.29,29.21 R1.1 19.47,30.01 19.94,30.48 25.02,30.48 v25.78,29.72 | v32.51,26.16 32.77,25.91 38.23,25.91 38.99,25.15 38.99,22.99 40.64,21.34 U4.40
  Bottom 0.254: v25.78,29.72 26.29,29.21 30.35,29.21 32.51,27.05 v32.51,26.16
SD_D2  (via drill 0.25, 0.51)
  Top 0.254: U4.51 45.93,26.12 45.72,25.91 v43.69,25.91 | 19.56,19.14 R5.1 12.83,19.05 v10.41,21.46 5.89,21.46 J3.1 | v18.16,30.99 18.41,31.24 35.69,31.24 37.21,29.72 41.66,29.72 42.16,29.21 v43.18,29.21
  Bottom 0.254: v18.16,30.99 17.91,30.99 15.24,33.66 12.45,33.66 10.54,31.75 10.54,21.59 v10.41,21.46 | v43.69,25.91 43.69,28.7 v43.18,29.21
SD_D3  (via drill 0.25, 0.51)
  Top 0.254: J3.2 11.78,22.64 v11.81,22.61 11.81,22.48 13.97,20.32 16.51,20.32 17.78,21.59 R4.1 19.56,21.68 | v42.55,30.23 37.72,30.23 36.07,31.88 16.13,31.88 v15.75,31.5 | v45.09,31.62 45.43,31.28 U4.52
  Bottom 0.254: v45.09,31.62 43.94,31.62 v42.55,30.23 | v15.75,31.5 15.75,31.62 14.48,32.89 12.7,32.89 11.81,32 v11.81,22.61
SPKR+  (via drill 0.51)
  Top 0.254: v55.88,43.18 55.88,49.78 56.52,50.42 U6.8
  Bottom 0.254: J5.2 57.15,41.91 v55.88,43.18
SPKR-
  Top 0.254: J5.1 60.96,40.64 60.96,42.55 62.23,43.81 62.23,50.04 61.98,50.29 61.17,50.29 R10.2 59.43,50.38 U6.5
TRIG00
  Top 0.254: U4.14 35.48,18.84 34.04,17.4 34.04,15.49 33.4,14.86 25.02,14.86 24.51,15.37 24.51,16.09 R40.2
TRIG01
  Top 0.254: U4.15 35.74,18.34 34.67,17.27 34.67,15.37 33.66,14.35 8.76,14.35 7.11,12.7 R39.2
TRIG02
  Top 0.254: U4.16 36,17.84 35.31,17.14 35.31,15.24 33.91,13.84 11.56,13.84 10.41,12.7 R38.2
TRIG03
  Top 0.254: R37.2 13.72,12.57 14.48,13.34 34.16,13.34 35.81,14.99 39.12,14.99 39.43,15.3 U4.17
TRIG04
  Top 0.254: U4.20 40.93,14.64 40.77,14.48 36.07,14.48 34.42,12.83 17.91,12.83 17.14,12.06 R36.2
TRIG05
  Top 0.254: U4.21 41.43,14.38 41.02,13.97 36.32,13.97 34.67,12.32 21.34,12.32 20.45,11.43 R35.2
TRIG06
  Top 0.254: U4.22 41.93,14.12 41.27,13.46 36.58,13.46 34.92,11.81 24.38,11.81 23.75,11.18 R34.2
TRIG07
  Top 0.254: U4.23 42.43,13.86 41.53,12.95 36.83,12.95 35.18,11.3 27.69,11.3 27.05,10.67 R33.2
TRIG08  (via drill 0.25)
  Top 0.254: U4.61 40.93,26.63 v41.91,25.65 | v30.48,9.02 30.48,9.27 30.99,9.78 31.71,9.78 R11.2
  Bottom 0.254: v41.91,25.65 41.91,24.13 42.8,23.24 42.8,18.67 41.91,17.78 37.85,17.78 37.59,17.53 37.59,14.73 36.32,13.46 34.42,13.46 31.75,10.79 31.75,10.29 v30.48,9.02
TRIG09  (via drill 0.25)
  Top 0.254: U4.62 40.43,26.12 v40.77,25.78 | 35.18,9.87 R12.2 35.05,10.41 34.67,10.79 30.86,10.79 v30.61,10.54
  Bottom 0.254: v40.77,25.78 40.77,24.51 42.29,22.99 42.29,18.92 41.66,18.29 37.34,18.29 37.08,18.03 37.08,15.24 35.94,14.1 34.16,14.1 v30.61,10.54
TRIG10  (via drill 0.25)
  Top 0.254: U4.29 45.43,14.89 46.1,14.22 47.5,14.22 48.26,13.46 v48.26,11.81 | R13.2 38.35,10.79 v38.48,10.92
  Bottom 0.254: v48.26,11.81 48.26,11.3 47.12,10.16 39.24,10.16 v38.48,10.92
TRIG11  (via drill 0.25)
  Top 0.254: U4.44 45.31,23.34 v44.83,22.86 | v41.66,11.05 R18.2
  Bottom 0.254: v41.66,11.05 42.42,11.05 45.09,13.72 45.09,22.61 v44.83,22.86
TRIG12  (via drill 0.25)
  Top 0.254: U4.45 45.88,23.84 v45.59,24.13 | v44.96,11.3 R21.2
  Bottom 0.254: v44.96,11.3 44.96,12.83 45.59,13.46 v45.59,24.13
TRIG13  (via drill 0.25)
  Top 0.254: U4.46 50.34,24.34 v50.67,24 | R22.2 48.26,10.67 49.15,11.56 49.15,12.32 50.04,13.21 v52.2,13.21
  Bottom 0.254: v50.67,24 50.67,23.75 50.16,23.24 50.16,16.76 50.8,16.13 50.8,14.61 v52.2,13.21
TRIG14  (via drill 0.25)
  Top 0.254: v47.5,28.96 47.24,28.96 46.93,28.64 U4.49 | v51.56,11.18 R23.2
  Bottom 0.254: v47.5,28.96 47.5,17.91 49.28,16.13 49.28,13.46 v51.56,11.18
TRIG15  (via drill 0.25, 0.51)
  Top 0.254: v48.51,29.84 48.01,30.35 47.12,30.35 46.43,29.67 U4.50 | v54.86,11.18 R24.2
  Bottom 0.254: v48.51,29.84 48.51,17.65 49.91,16.26 49.91,14.22 52.2,11.94 54.1,11.94 v54.86,11.18
TXD  (via drill 0.51)
  Top 0.254: v52.07,21.84 50.93,21.84 50.43,22.34 U4.42 | v58.42,19.18 58.42,13.97 J4.5
  Bottom 0.254: v58.42,19.18 58.29,19.18 56.64,20.83 53.09,20.83 v52.07,21.84
VCC  (via drill 0.25, 0.51)
  Top 0.203: R29.2 43.98,9.74 44.13,9.65 v44.13,5.97 | v40.83,5.97 40.83,9.53 40.7,9.65 40.09,9.65 R30.2 | R31.2 37.44,9.74 37.53,9.65 v37.53,6.73 | R32.2 34.14,9.74 34.23,9.65 v34.23,6.73
  Top 0.254: 40.51,46.61 41.02,47.12 U5.1 41.02,49.91 43.18,52.07 C21.2 | 36.45,47.12 36.45,48.59 U5.8 36.48,51.16 35.56,52.07 C27.2 34.89,53.76 33.66,54.99 SJ4.1 SJ4.2 29.34,54.99 28.96,54.61 28.96,53.98 28.32,53.34 C5.1 v27.56,51.82 | 36.45,47.12 35.47,46.14 C26.2 C22.1 | U5.20 41.02,46.1 40.51,46.61 | 23.75,38.48 24.13,38.1 28.03,38.1 28.79,38.86 | 23.75,38.48 23.75,39.33 C11.1 | 20.83,35.56 R17.1 18.67,35.52 18.67,34.67 18.41,34.42 10.29,34.42 8.76,32.89 5.59,32.89 4.06,31.37 1.78,31.37 1.4,30.99 1.4,26.04 2.67,24.77 4.06,24.77 | 20.83,35.56 23.75,38.48 | R5.2 R4.2 R3.2 R2.2 R1.2 v22.86,29.21 | v5.46,18.67 3.81,20.32 3.81,24.51 4.06,24.77 | J3.4 5.54,24.77 4.06,24.77 | 20.83,35.56 21.59,35.56 v22.1,35.05 | 28.79,38.86 C19.1 28.79,43.81 28.57,44.03 C12.1 27.94,45.21 27.62,45.53 U2.5 28.55,46.96 28.96,47.37 28.96,49.28 v28.83,49.4 | 28.79,38.86 v28.79,34.96 | v29.97,30.1 30.23,30.1 32.38,27.94 C18.1 35.18,27.9 35.18,27.3 35.43,27.05 38.48,27.05 38.77,27.34 U4.64 39.43,26.36 39.88,25.91 39.88,25.65 40.77,24.77 40.77,24.64 | 40.77,24.64 40.77,23.24 v41.27,22.73 | 40.77,24.64 41.02,24.89 43.94,24.89 44.39,25.34 U4.48 49.85,25.34 50.29,25.78 | v39.24,19.05 38.35,19.05 38.06,19.34 U4.13 34.58,19.34 34.04,18.8 33.27,18.8 33.02,18.54 C13.1 | v49.53,27.94 49.53,26.54 50.29,25.78 | 50.29,25.78 51.02,25.78 C10.1 | R29.2 C9.1 43.98,11.47 44.7,12.19 v45.85,12.19 45.85,10.92 46.61,10.16 R28.2 | R26.2 53.21,10.41 52.83,10.79 52.83,12.7 | 52.83,12.7 53.21,13.08 53.59,13.08 53.72,13.21 53.72,13.93 R19.1 53.76,14.99 | 53.76,14.99 R14.2 53.21,15.88 52.45,16.64 49.28,16.64 49.15,16.51 49.15,15.79 C15.1 49.12,15.68 48.26,15.68 v48.01,15.43 47.82,15.24 46.99,15.24 46.93,15.3 U4.32 46.93,17.2 45.21,18.92 42.04,18.92 41.91,19.05 v41.4,19.05 41.4,17.78 40.43,16.81 U4.19
  Top 0.254: v8.76,11.18 R47.2 | R46.2 v12.06,11.18 | R45.2 v15.37,11.18 | R44.2 v18.8,11.18 | R43.2 v22.1,11.18 | R42.2 v25.4,10.92 | v29.72,7.11 29.72,9.4 29.34,9.78 28.74,9.78 R41.2 | R25.2 56.52,14.61 56.26,14.86 53.89,14.86 53.76,14.99 | R27.2 49.91,11.3 50.67,12.06 52.2,12.06 52.83,12.7 | 36.45,47.12 36.45,46.86 36.83,46.48 40.39,46.48 40.51,46.61 | R48.2 v16.76,16.13
  Bottom 0.203: v44.13,5.97 v40.83,5.97 38.29,5.97 v37.53,6.73 v34.23,6.73
  Bottom 0.254: v49.53,27.94 57.15,27.94 58.42,29.21 60.96,29.21 J8.3 | v22.86,29.21 22.86,34.29 v22.1,35.05 | 29.84,30.23 v29.97,30.1 29.97,33.27 28.79,34.46 v28.79,34.96 | v39.24,19.05 v41.4,19.05 41.66,19.3 41.66,20.19 41.27,20.57 v41.27,22.73 | v45.85,12.19 47.24,12.19 48.01,12.95 v48.01,15.43 48.26,15.68 | v15.37,11.18 v12.06,11.18 v8.76,11.18 8.76,15.37 v5.46,18.67 | v15.37,11.18 v18.8,11.18 v22.1,11.18 25.15,11.18 v25.4,10.92 25.91,10.92 26.29,10.54 26.29,7.37 26.8,6.86 29.46,6.86 v29.72,7.11 | v28.83,49.4 28.83,50.55 v27.56,51.82 | v16.76,16.13 16.76,12.57 v15.37,11.18
VIN
  Top 0.254: J1.VIN0 3.81,48.51 4.32,48.01 | 4.32,48.01 14.48,48.01 | 14.48,48.01 15.75,49.28 15.75,51.33 U1.3 | J9.2 1.27,44.96 4.32,48.01 | C1.1 15.24,39.37 14.48,40.13 12.7,41.91 12.7,46.23 14.48,48.01

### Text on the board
Bottom: v11
tPlace: LOAD | RUN | + | SPKR | - | WAV Trigger | 5V | VIN | GND | robertsonics | LR | 5V | BC | 3.3V | DI | PLO | MC | GND | I2S | BLK | GND | 5Vin | LED | RX | TX | T1 | T1 | T2 | T3 | T4 | T5 | T6 | T7 | T8 | T9 | T10 | T11 | T12 | T13 | T14 | T15 | T16 | GRN | GND | GND | Triggers | Triggers
bPlace: WAV Trigger
tNames: Jamie Robertson, Jordan McConnell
